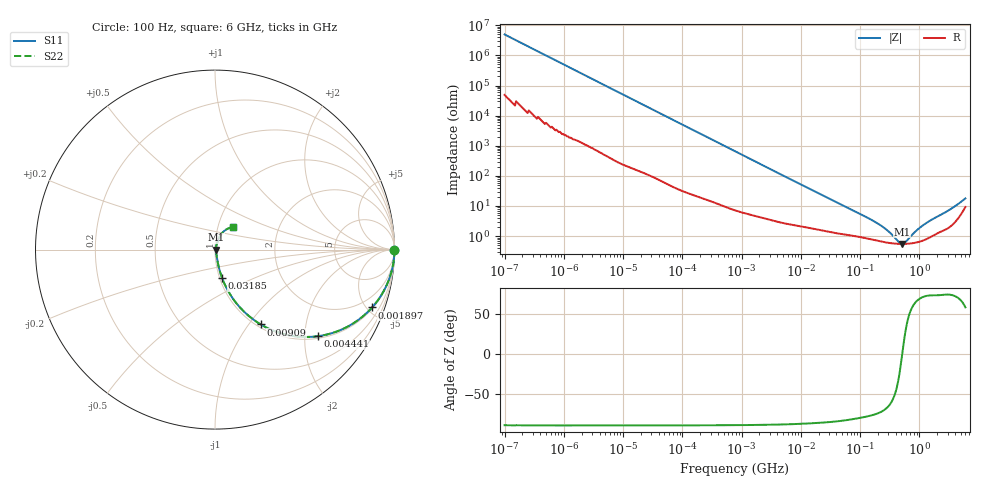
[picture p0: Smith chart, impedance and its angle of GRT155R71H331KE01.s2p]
!Murata Part Number: GRT155R71H331KE01
!These Parameters are Measured in Series Mode Connection
!Data Generated on Jun 19, 2026
!  o--ll--o
!Port1  Port2
!  o------o
!Operation Temp=25[degC], DC Bias Voltage=0[V]
!Freq. Start=100[Hz] Stop=6[GHz] 401[Steps]
# Hz S RI R 50
!Freq.(Hz) S11(Real) S11(Imag) S21(Real) S21(Imag) S12(Real) S12(Imag) S22(Real) S22(Imag)
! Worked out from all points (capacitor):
!   401 points, 100 Hz to 6 GHz, reference 50 ohm
!   read as one part in series: C = 322 pF near 109 Hz
!   lowest |Z| = 553 mohm at 511.3 MHz (marker M1)
!   series resonance near 514.9 MHz, so ESL is about 300 pH
!   S11 on the Smith chart (normalised r, x): 100 Hz: open; 1.897 MHz: 1.09, -5.40; 4.441 MHz: 1.06, -2.32; 9.09 MHz: 1.04, -1.14; 31.85 MHz: 1.03, -0.33; 6 GHz: 1.19, +0.31
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100  1 -2.02e-05  2e-07 2.02e-05  2e-07 2.02e-05  1 -2.02e-05
501  1 -0.000101  6e-07 0.000101  6e-07 0.000101  1 -0.000101
2008  1 -0.000403  2.2e-06 0.000403  2.2e-06 0.000403  1 -0.000403
40335  0.9999 -0.00802  0.000112 0.00802  0.000112 0.00802  0.9999 -0.00802
241822  0.9973 -0.0476  0.00266 0.0476  0.00266 0.0476  0.9973 -0.0476
774597  0.9758 -0.1482  0.0242 0.1482  0.0242 0.1482  0.9758 -0.1482
1896632  0.8754 -0.3222  0.1246 0.3222  0.1246 0.3222  0.8754 -0.3222
2837864  0.7619 -0.4162  0.2381 0.4162  0.2381 0.4162  0.7619 -0.4162
4440638  0.5726 -0.4825  0.4274 0.4825  0.4274 0.4825  0.5726 -0.4825
6353432  0.402 -0.4753  0.598 0.4753  0.598 0.4753  0.402 -0.4753
9090158  0.2548 -0.4171  0.7452 0.4171  0.7452 0.4171  0.2548 -0.4171
1.555665e7  0.1149 -0.2934  0.8851 0.2934  0.8851 0.2934  0.1149 -0.2934
3.184506e7  0.0395 -0.1586  0.9605 0.1586  0.9605 0.1586  0.0395 -0.1586
1.596157e8  0.00871 -0.0325  0.9913 0.0325  0.9913 0.0325  0.00871 -0.0325
3.124326e8  0.00606 -0.0121  0.9939 0.0121  0.9939 0.0121  0.00606 -0.0121
4.470121e8  0.00554 -0.00335  0.9945 0.00335  0.9945 0.00335  0.00554 -0.00335
5.112761e8  0.0055 -0.000165  0.9945 0.000165  0.9945 0.000165  0.0055 -0.000165
5.847788e8  0.00553 0.00304  0.9945 -0.00304  0.9945 -0.00304  0.00553 0.00304
8.749838e8  0.00625 0.0133  0.9937 -0.0133  0.9937 -0.0133  0.00625 0.0133
1.251881e9  0.00814 0.0241  0.9919 -0.0241  0.9919 -0.0241  0.00814 0.0241
3.666503e9  0.0304 0.08  0.9696 -0.08  0.9696 -0.08  0.0304 0.08
6e9  0.1025 0.1256  0.8975 -0.1256  0.8975 -0.1256  0.1025 0.1256
